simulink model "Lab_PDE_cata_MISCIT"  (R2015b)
settings: Solver=FixedStepAuto  StartTime=0.0  StopTime=Tsim  FixedStep=dt  RelTol=1e-3
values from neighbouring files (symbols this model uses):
  alpha_g = m_dot/(Aw_cat*rho_g)    (= 2.9867218971)    [init_lab_PDE.m]
  alpha_w = lambda_w/(rho_w*Cp_w)    (= 5.76923076923e-07)    [init_lab_PDE.m]
  beta_g = hi*Pi_cat/(Aw_cat*rho_g*Cp_g)    (= 8661.26213909)    [init_lab_PDE.m]
  beta_w = hi*Pi_cat/(Aw_cat*rho_w*Cp_w)    (= 3.92571706454)    [init_lab_PDE.m]
  dt = .01    (= 0.01)    [init_lab_PDE.m]
  dx = L/(N-1)    (= 0.002308)    [init_lab_PDE.m]
  epsilon = dx    (= 0.002308)    [init_lab_PDE.m]
  gamma_w = 1/(Aw_cat*rho_w*Cp_w)    (= 0.000140720550921)    [init_lab_PDE.m]
  N = 51    [init_lab_PDE.m]
  Tg_init = 20*ones(N,1)    [init_lab_PDE.m]
  Tw_init = 20*ones(N,1)    [init_lab_PDE.m]
  x0 = 20*dx    (= 0.04616)    [init_lab_PDE.m]

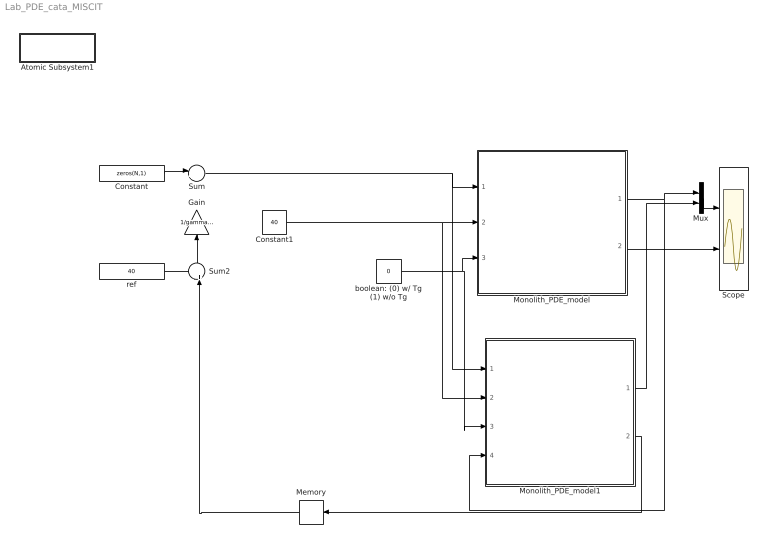
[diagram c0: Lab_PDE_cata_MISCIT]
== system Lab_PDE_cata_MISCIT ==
  Atomic Subsystem1 : Subsystem
  Constant : Constant  Value=zeros(N,1)
  Constant1 : Constant  Value=40
  Gain : Gain  Gain=1/gamma_w
  Memory : Memory  X0=Tw_init
  Monolith_PDE_model : Subsystem  TreatAsAtomicUnit=on
  Monolith_PDE_model1 : Subsystem  TreatAsAtomicUnit=on
  Mux : Mux  Inputs=2
  Scope : Scope  NumInputPorts=2
  Sum : Sum  Inputs=|+-
  Sum2 : Sum  Inputs=-+|
  boolean: (0) w/ Tg (1) w/o Tg : Constant  Value=0
  ref : Constant  Value=40
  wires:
  Monolith_PDE_model/1(Tw_x0) -> Mux/1, Monolith_PDE_model1/4(Tw_x0)
  Monolith_PDE_model/2(Tg_L) -> Scope/2
  boolean: (0) w/ Tg (1) w/o Tg/1 -> Monolith_PDE_model1/3(boolean), Monolith_PDE_model/3(boolean)
  Monolith_PDE_model1/1(Tw_x0_hat) -> Mux/2
  Mux/1 -> Scope/1
  Sum/1 -> Monolith_PDE_model1/1(f), Monolith_PDE_model/1(f)
  Constant/1 -> Sum/1
  Sum2/1 -> Gain/1
  ref/1 -> Sum2/1
  Monolith_PDE_model1/2(Tw_hat) -> Memory/1
  Memory/1 -> Sum2/2
  Constant1/1 -> Monolith_PDE_model1/2(Tg0), Monolith_PDE_model/2(Tg0)

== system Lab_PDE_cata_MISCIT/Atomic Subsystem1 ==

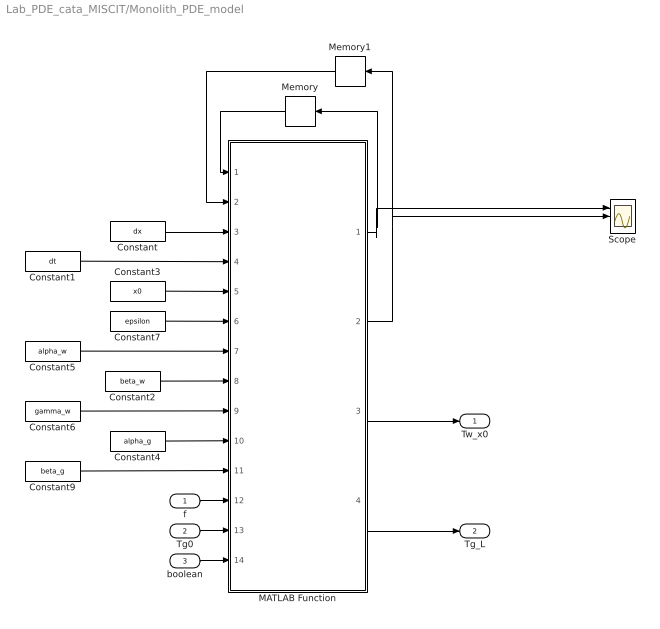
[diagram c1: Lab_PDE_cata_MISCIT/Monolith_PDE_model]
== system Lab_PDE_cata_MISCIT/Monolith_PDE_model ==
  f : Inport
  Tg0 : Inport  Port=2
  boolean : Inport  Port=3
  Constant : Constant  Value=dx
  Constant1 : Constant  Value=dt
  Constant2 : Constant  Value=beta_w
  Constant3 : Constant  Value=x0
  Constant4 : Constant  Value=alpha_g
  Constant5 : Constant  Value=alpha_w
  Constant6 : Constant  Value=gamma_w
  Constant7 : Constant  Value=epsilon
  Constant9 : Constant  Value=beta_g
  MATLAB Function : MATLAB Function  TreatAsAtomicUnit=on
  Memory : Memory  X0=Tw_init
  Memory1 : Memory  X0=Tg_init
  Scope : Scope  NumInputPorts=3
  Tw_x0 : Outport
  Tg_L : Outport  Port=2
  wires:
  Constant/1 -> MATLAB Function/3(dx)
  Constant1/1 -> MATLAB Function/4(dt)
  Memory/1 -> MATLAB Function/1(u)
  MATLAB Function/1(u1) -> Memory/1, Scope/1
  MATLAB Function/2(v1) -> Scope/2, Memory1/1
  Tg0/1 -> MATLAB Function/13(Tgin)
  Memory1/1 -> MATLAB Function/2(v)
  MATLAB Function/4(Tgout) -> Tg_L/1
  Constant5/1 -> MATLAB Function/7(alpha_w)
  Constant6/1 -> MATLAB Function/9(gamma_w)
  Constant9/1 -> MATLAB Function/11(beta_g)
  Constant2/1 -> MATLAB Function/8(beta_w)
  Constant4/1 -> MATLAB Function/10(alpha_g)
  f/1 -> MATLAB Function/12(f)
  Constant3/1 -> MATLAB Function/5(x0)
  Constant7/1 -> MATLAB Function/6(epsilon)
  MATLAB Function/3(Twx0) -> Tw_x0/1
  boolean/1 -> MATLAB Function/14(boolean)

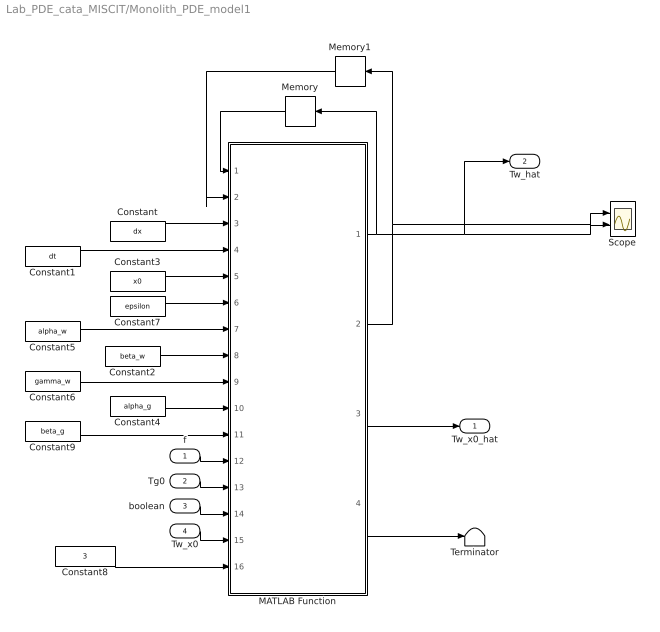
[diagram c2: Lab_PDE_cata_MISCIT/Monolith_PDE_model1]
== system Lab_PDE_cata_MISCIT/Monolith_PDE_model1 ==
  f : Inport
  Tg0 : Inport  Port=2
  boolean : Inport  Port=3
  Tw_x0 : Inport  Port=4
  Constant : Constant  Value=dx
  Constant1 : Constant  Value=dt
  Constant2 : Constant  Value=beta_w
  Constant3 : Constant  Value=x0
  Constant4 : Constant  Value=alpha_g
  Constant5 : Constant  Value=alpha_w
  Constant6 : Constant  Value=gamma_w
  Constant7 : Constant  Value=epsilon
  Constant8 : Constant  Value=3
  Constant9 : Constant  Value=beta_g
  MATLAB Function : MATLAB Function  TreatAsAtomicUnit=on
  Memory : Memory  X0=zeros(N,1)
  Memory1 : Memory  X0=zeros(N,1)
  Scope : Scope  NumInputPorts=2
  Terminator : Terminator
  Tw_x0_hat : Outport
  Tw_hat : Outport  Port=2
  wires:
  Constant/1 -> MATLAB Function/3(dx)
  Constant1/1 -> MATLAB Function/4(dt)
  Memory/1 -> MATLAB Function/1(u)
  MATLAB Function/1(u1) -> Memory/1, Tw_hat/1, Scope/1
  MATLAB Function/2(v1) -> Scope/2, Memory1/1
  Tg0/1 -> MATLAB Function/13(Tgin)
  Memory1/1 -> MATLAB Function/2(v)
  MATLAB Function/4(Tgout) -> Terminator/1
  Constant5/1 -> MATLAB Function/7(alpha_w)
  Constant6/1 -> MATLAB Function/9(gamma_w)
  Constant9/1 -> MATLAB Function/11(beta_g)
  Constant2/1 -> MATLAB Function/8(beta_w)
  Constant4/1 -> MATLAB Function/10(alpha_g)
  f/1 -> MATLAB Function/12(f)
  Constant3/1 -> MATLAB Function/5(x0)
  Constant7/1 -> MATLAB Function/6(epsilon)
  MATLAB Function/3(Twx0) -> Tw_x0_hat/1
  boolean/1 -> MATLAB Function/14(boolean)
  Tw_x0/1 -> MATLAB Function/15(y)
  Constant8/1 -> MATLAB Function/16(l)

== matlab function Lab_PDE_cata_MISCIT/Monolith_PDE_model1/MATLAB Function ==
function [u1,v1,Twx0,Tgout] = fcn(u,v,dx,dt,x0,epsilon,alpha_w,beta_w,gamma_w,alpha_g,beta_g,f,Tgin,boolean,y,l)

N = 51;

% Dynamics matrices -- Implicit scheme
A1 = eye(N)*(1+2*alpha_w*dt/dx^2+beta_w*dt) + diag(-alpha_w*dt/dx^2*ones(1,N-1),-1) + diag(-alpha_w*dt/dx^2*ones(1,N-1),1) ;
A2 = -beta_w*dt*eye(N);
A3 = -beta_g*dt*eye(N);
A4 = eye(N)*(1+alpha_g*dt/dx+beta_g*dt) + diag(-alpha_g*dt/dx*ones(1,N-1),-1);
A = [A1 A2; A3 A4];

% Boundary conditions
A(1,:) = [1+2*alpha_w*dt/dx^2+beta_w*dt -2*alpha_w*dt/dx^2 zeros(1,N-2) -beta_w*dt zeros(1,N-1)];
A(N,:) = [zeros(1,N-2) -2*alpha_w*dt/dx^2 1+2*alpha_w*dt/dx^2+beta_w*dt zeros(1,N-1) -beta_w*dt];
A(N+1,:) = [zeros(1,N) 1 zeros(1,N-1)];
B1 = eye(2*N);
B1(N+1,:) = zeros(1,2*N);
B2 = zeros(2*N,1);
B2(N+1,:) = 1;

int_x0 = round(x0/dx);
int_epsilon = round(epsilon/dx);
Twx0_hat = dx/(2*epsilon)*sum(u(int_x0-int_epsilon:int_x0+int_epsilon-1));

% Dynamics
X = zeros(2*N,1);
X = inv(A)*(B1*[u;v] + B2*Tgin + [dt*gamma_w*f;zeros(N,1)] + [l*dt*(y-Twx0_hat)*ones(N,1); zeros(N,1)] );
u1 = X(1:N);
v1 = X(N+1:end);

if boolean == 1
    v1 = v;
end

int_x0 = round(x0/dx);
int_epsilon = round(epsilon/dx);
Twx0 = dx/(2*epsilon)*sum(u1(int_x0-int_epsilon:int_x0+int_epsilon-1));
Tgout = v1(end);

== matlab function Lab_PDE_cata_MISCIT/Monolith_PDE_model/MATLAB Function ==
function [u1,v1,Twx0,Tgout] = fcn(u,v,dx,dt,x0,epsilon,alpha_w,beta_w,gamma_w,alpha_g,beta_g,f,Tgin,boolean)

N = 51;

% Dynamics matrices -- Implicit scheme
A1 = eye(N)*(1+2*alpha_w*dt/dx^2+beta_w*dt) + diag(-alpha_w*dt/dx^2*ones(1,N-1),-1) + diag(-alpha_w*dt/dx^2*ones(1,N-1),1) ;
A2 = -beta_w*dt*eye(N);
A3 = -beta_g*dt*eye(N);
A4 = eye(N)*(1+alpha_g*dt/dx+beta_g*dt) + diag(-alpha_g*dt/dx*ones(1,N-1),-1);
A = [A1 A2; A3 A4];

% Boundary conditions
A(1,:) = [1+2*alpha_w*dt/dx^2+beta_w*dt -2*alpha_w*dt/dx^2 zeros(1,N-2) -beta_w*dt zeros(1,N-1)];
A(N,:) = [zeros(1,N-2) -2*alpha_w*dt/dx^2 1+2*alpha_w*dt/dx^2+beta_w*dt zeros(1,N-1) -beta_w*dt];
A(N+1,:) = [zeros(1,N) 1 zeros(1,N-1)];
B1 = eye(2*N);
B1(N+1,:) = zeros(1,2*N);
B2 = zeros(2*N,1);
B2(N+1,:) = 1;

% Dynamics
X = zeros(2*N,1);
X = inv(A)*(B1*[u;v] + B2*Tgin + [dt*gamma_w*f;zeros(N,1)] );
u1 = X(1:N);
v1 = X(N+1:end);

if boolean == 1
    v1 = v;
end

int_x0 = round(x0/dx);
int_epsilon = round(epsilon/dx);
Twx0 = dx/(2*epsilon)*sum(u1(int_x0-int_epsilon:int_x0+int_epsilon-1));
Tgout = v1(end);
